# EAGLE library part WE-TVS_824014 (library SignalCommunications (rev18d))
TVS Diode Super Speed Series Characteristics Operating temperature: –55 ºC to +85 °C for 824 014 x; –40 ºC to +85 °C for 824 016 46 Low clamping voltage Very low capacitance Rail to Rail protection Epoxy flame resistant UL94 V-0 RoHS, REACH and free of halogens Applications Super Speed data lines HDMI 1.3/1.4, DVI DisplayPort USB 3.0 SuperSpeed SATA GBit LAN ESD protection in accordance with EN 61000-4-2 – 8 kV contact discharge – 15 kV air discharge Details see: http://katalog.we-online.de/en/pbs/WE-TVS_High_Speed/24014? Updated by Dan Xu 2014-07-11 2014 (C) Wurth Elektronik
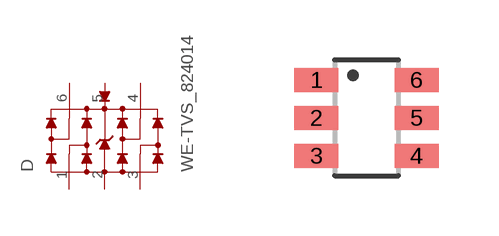
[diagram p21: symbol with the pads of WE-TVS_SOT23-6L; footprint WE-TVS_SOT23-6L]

Designator prefix D

## WE-TVS_824014  [WE-TVS_SOT23-6L]
1  1  pas
2  GND  pwr
3  2  pas
4  3  pas
5  VDD  pwr
6  4  pas

## Footprint WE-TVS_SOT23-6L (pad centres in mm)
TVS Diode Array WE-TVS
smd 1.1 x 0.6: 1 -1.25,0.95; 2 -1.25,0; 3 -1.25,-0.95; 4 1.25,-0.95; 5 1.25,0; 6 1.25,0.95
